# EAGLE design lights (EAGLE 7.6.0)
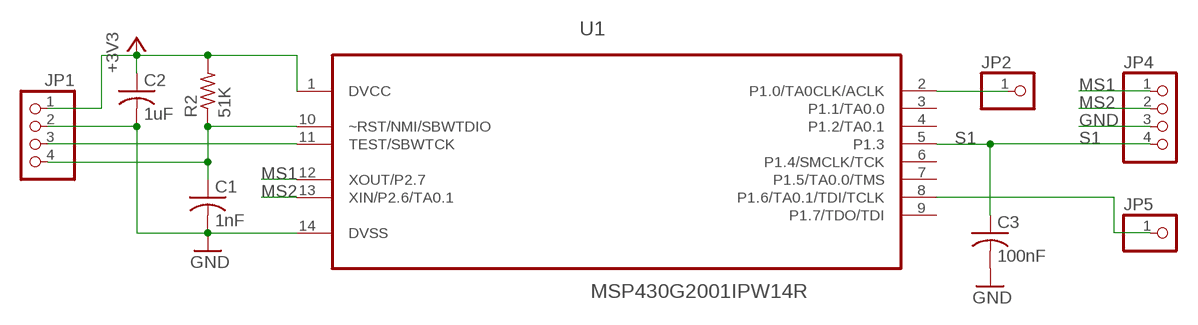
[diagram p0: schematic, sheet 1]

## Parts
C1  1nF  C-USC1206  [C1206]
C2  1uF  C-USC1206  [C1206]
C3  100nF  C-USC1206  [C1206]
JP1  PINHD-1X4  [1X04]
JP2  PINHD-1X1  [1X01]
JP4  PINHD-1X4  [1X04]
JP5  PINHD-1X1  [1X01]
R2  51K  R-US_0204/7  [0204/7]
U1  MSP430G2001IPW14R  [SOP65P640X120-14N]

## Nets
+3V3: C2.1 JP1.1 R2.2 U1.1(DVCC)
GND: C1.2 C2.2 C3.2 JP1.2 JP4.3 U1.14(DVSS)
MS1: JP4.1 U1.12(XOUT/P2.7)
MS2: JP4.2 U1.13(XIN/P2.6/TA0.1)
N$1: C1.1 JP1.4 R2.1 U1.10(~RST/NMI/SBWTDIO)
N$2: JP1.3 U1.11(TEST/SBWTCK)
N$3: JP2.1 U1.2(P1.0/TA0CLK/ACLK)
N$4: JP5.1 U1.8(P1.6/TA0.1/TDI/TCLK)
S1: C3.1 JP4.4 U1.5(P1.3)
Unconnected: U1.3(P1.1/TA0.0) U1.4(P1.2/TA0.1) U1.6(P1.4/SMCLK/TCK) U1.7(P1.5/TA0.0/TMS) U1.9(P1.7/TDO/TDI)

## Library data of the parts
C1-C3 = resistor:C-US: CAPACITOR, American symbol
JP1 JP4 = pinhead:PINHD-1X4: PIN HEADER
JP2 JP5 = pinhead:PINHD-1X1: PIN HEADER
R2 = resistor:R-US_: RESISTOR, American symbol
U1 = custom:MSP430G2001IPW14R: MIXED SIGNAL MICROCONTROLLER; MPN: MSP430G2001IPW14R; OC_FARNELL: -; OC_NEWARK: 74R6476; PACKAGE: TSSOP-14; SUPPLIER: Texas Instruments

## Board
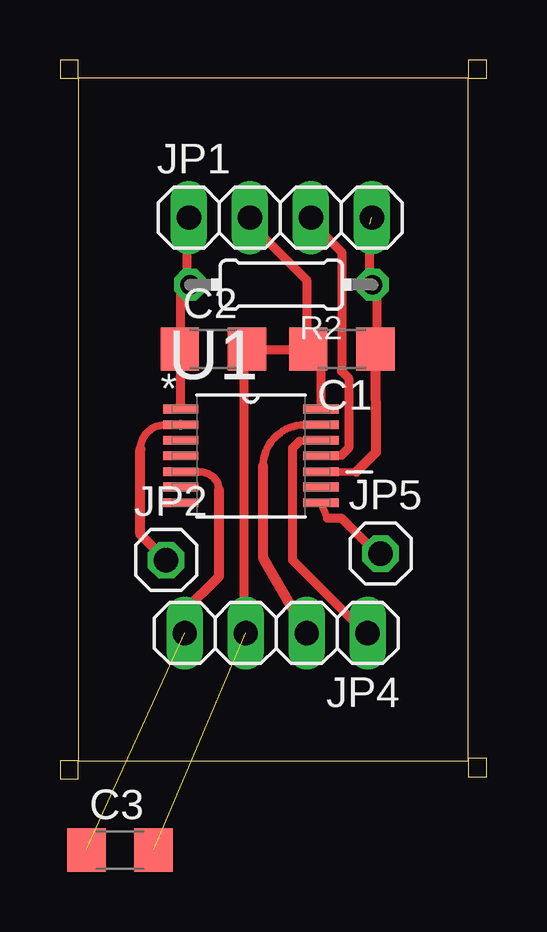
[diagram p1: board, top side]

Size 17.78 x 29.97 mm. Coordinates in mm from the lower left corner, seen from the top.
Outline: 0.76,0.76 17.02,0.76 17.02,29.21 0.76,29.21 0.76,0.76
Copper layers (1*16): Top 0.035mm / dielectric 1.5mm / Bottom 0.035mm
Design rules "default *": minimum track width 15mil, minimum drill 1mil, track to track 8mil, track to pad 8mil, pad to pad 8mil, via to via 8mil, smd to smd 8mil, copper to edge 40mil, drill to drill 8mil, minimum pad ring 10mil, minimum via ring 8mil, stop-mask expansion 4mil, vias tented up to drill 0mil, thermal gap 10mil

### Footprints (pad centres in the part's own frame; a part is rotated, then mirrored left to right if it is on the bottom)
C1206 = smd 1.6 x 1.8: 1 -1.4,0; 2 1.4,0
1X04 = drill 1.016 long: 1 -3.81,0; 2 -1.27,0; 3 1.27,0; 4 3.81,0
1X01 = drill 1.016 octagon: 1 0,0
0204/7 = drill 0.813 octagon: 1 -3.81,0; 2 3.81,0
SOP65P640X120-14N = smd 1.473 x 0.356: 1 -2.921,1.956; 2 -2.921,1.295; 3 -2.921,0.66; 4 -2.921,0; 5 -2.921,-0.66; 6 -2.921,-1.295; 7 -2.921,-1.956; 8 2.921,-1.956; 9 2.921,-1.295; 10 2.921,-0.66; 11 2.921,0; 12 2.921,0.66; 13 2.921,1.295; 14 2.921,1.956

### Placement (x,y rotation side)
C1  11.74,17.91 180 top
C2  6.39,17.92 0 top
C3  2.5,-2.96 0 top
JP1  9.18,23.4 0 top
JP2  4.42,9.12 0 top
JP4  9.01,6.08 180 top
JP5  13.36,9.39 0 top
R2  9.22,20.61 180 top
U1  7.95,13.46 0 top

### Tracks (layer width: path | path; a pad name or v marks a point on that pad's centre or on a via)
+3V3
  Top 0.381: JP1.1 5.31,23.13 5.31,20.8 R2.2 5.02,20.21 5.02,18.17 C2.1 5.02,17.88 5.02,15.54 U1.1
GND  (1 unrouted)
  Top 0.381: 10.86,17.58 10.57,17.88 C1.2 | C1.2 10.27,18.17 10.27,20.8 7.94,23.13 JP1.2 | 10.86,17.58 10.86,15.54 U1.14 | 10.86,17.58 C1.2 | C1.2 10.27,17.88 7.94,17.88 C2.2 7.65,17.88 7.65,6.19 JP4.3
MS1
  Top 0.305: 9.98,14.08 10.86,14.08 U1.12
  Top 0.381: 9.98,14.08 9.69,13.79 9.69,9.11 12.61,6.19 JP4.1
MS2
  Top 0.305: 8.46,13.03 arc-90 10.19,14.76 U1.13 arc90 U1.13
  Top 0.406: JP4.2 8.46,9.2 8.46,13.03
N$1  (1 unrouted)
  Top 0.305: 12.35,12.8 U1.10
  Top 0.381: C1.1 13.2,18.17 13.2,20.5 R2.1 12.9,20.8 12.9,23.13
  Top 0.406: C1.1 13.16,13.61 12.35,12.8
N$2
  Top 0.305: 11.74,13.49 11.15,13.49 U1.11
  Top 0.381: JP1.3 10.57,23.13 11.74,21.97 11.74,17 12.03,16.71 12.03,13.79 11.74,13.49
N$3
  Top 0.305: 3.35,13.74 arc-90 4.37,14.76 U1.2
  Top 0.406: JP2.1 3.35,10.19 3.35,13.74 | U1.2 arc90 U1.2
N$4
  Top 0.305: 11.15,10.87 U1.8
  Top 0.381: 11.15,10.87 11.74,10.87 13.2,9.41 JP5.1
S1  (1 unrouted)
  Top 0.305: 6.62,12.04 arc90 5.87,12.79 5.05,12.79 arc-90 U1.5
  Top 0.406: JP4.4 5.2,7.02 6.62,8.45 6.62,12.04

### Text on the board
Document: +0TR | L | L | B0MM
